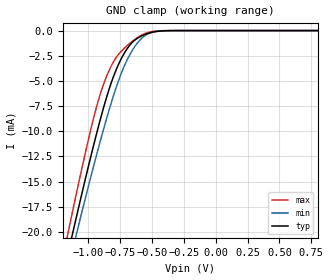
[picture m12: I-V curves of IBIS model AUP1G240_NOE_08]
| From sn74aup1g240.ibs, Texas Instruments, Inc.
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[Model]   AUP1G240_NOE_08
Model_type  Input
Vinl=0
Vinh=0.8
| variable   typ   min   max
C_comp   1.71pF   1.55pF   1.90pF
[Temperature Range]   40   100   -40
| Ambient temperature   25   85   -40
[Voltage range]   0.8   0.8   0.8
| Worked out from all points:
|   GND clamp passes 1 mA (typ) near -0.64 V on its own axis
[GND Clamp]
| AUP1G240_NOE_08
|   Voltage   I(typ)   I(min)   I(max)
-3.6V     -171.6mA   -163.5mA   -181.1mA
-1.165V   -22.5mA    -23.95mA   -20.48mA
-1.12V    -20mA      -21.61mA   -17.78mA
-1.1V     -18.9mA    -20.58mA   -16.6mA
-1.08V    -17.81mA   -19.55mA   -15.42mA
-955mV    -11.25mA   -13.33mA   -8.55mA
-855mV    -6.58mA    -8.69mA    -4.512mA
-790mV    -4.17mA    -5.995mA   -2.849mA
-720mV    -2.308mA   -3.6mA     -1.791mA
-575mV    -491.1uA   -700uA     -410.3uA
-400mV    -19.26uA   -24.01uA   -5.501uA
800mV     56.96pA    394.1pA    9.079pA
